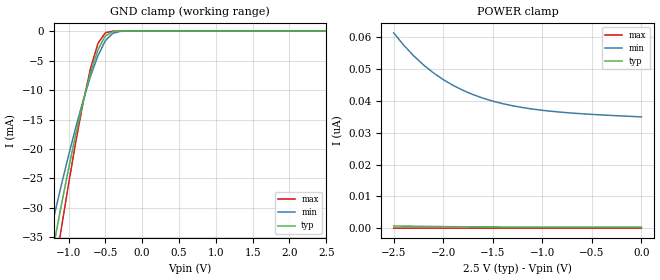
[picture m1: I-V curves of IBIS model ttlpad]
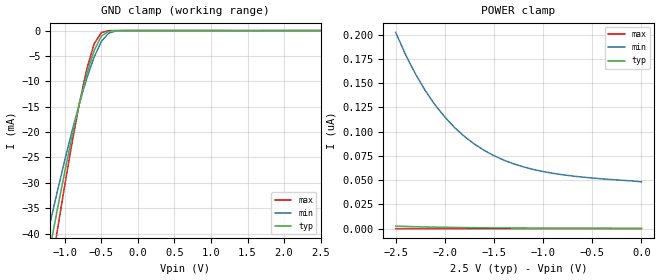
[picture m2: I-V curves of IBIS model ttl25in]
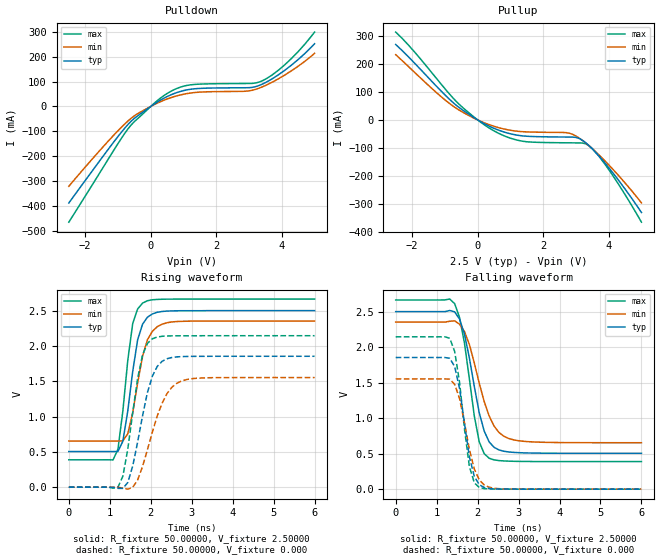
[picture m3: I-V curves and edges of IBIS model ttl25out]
| IBIS file idt45t9050.ibs created by s2ibis2 version 1.2
| North Carolina State University Electronics Research Laboratory  1995
[IBIS ver]   3.2
[File name]   idt45t9050.ibs
[File Rev]   1.0
[Date]   Friday, November 09, 2001
[Source]   Integrated Device Technology, Inc.
[Notes]
[Disclaimer] Integrated Device Technology, Inc. ("IDT") hereby grants the
   user of this IBIS model a non-exclusive, nontransferable
   license to use this IBIS model under the following terms. The
   user is granted this license only to use the IBIS model and is
   not granted rights to sell, copy (except as needed to run the
   IBIS model), rent, lease or sub-license the IBIS model in
   whole or in part, or in modified form to anyone. The User may
   modify the IBIS model to suit its specific applications, but
   rights to derivative works and such modifications shall belong
   to IDT. This IBIS model is provided on an AS IS" basis and IDT
   makes absolutely no warranty with respect to the information
   contained herein. IDT DISCLAIMS AND CUSTOMER WAIVES ALL
   WARRANTIES, EXPRESS AND IMPLIED, INCLUDING WARRANTIES OF
   MERCHANTABILITY AND FITNESS FOR A PARTICULAR PURPOSE. THE
   ENTIRE RISK AS TO QUALITY AND PERFORMANCE IS WITH THE USER
   ACCORDINGLY, IN NO EVENT SHALL IDT BE LIABLE FOR ANY DIRECT OR
   INDIRECT DAMAGES, WHETHER IN CONTRACT OR TORT, INCLUDING ANY
   LOST PROFITS OR OTHER INCIDENTAL, CONSEQUENTIAL, EXEMPLARY, OR
   PUNITIVE DAMAGES ARISING OUT OF THE USE OR APPLICATION OF THE
   IBIS model. Further, IDT reserves the right to make changes
   without notice to any product herein to improve reliability,
   function, or design. IDT does not convey any license under
   patent rights or any other intellectual property rights,
   including those of third parties. IDT is not obligated to
   provide maintenance or support for the licensed IBIS model.
[Copyright]   Copyright 2001, Integrated Device Technology, Inc. all rights
   reserved
|   Component idt45t9050
[Component]   idt45t9050
[Manufacturer]   Integrated Device Technology
|Package   PG28
[Package]
| variable   typ   min   max
R_pkg   2.40000m   2.40000m   2.40000m
L_pkg   0.90000nH   0.90000nH   0.90000nH
C_pkg   60.0000fF   60.0000fF   60.0000fF
[Pin]  signal_name   model_name   R_pin   L_pin   C_pin
1   GL   ttlpad
2   VDD   POWER
3   GND   GND
4   GX   ttlpad
5   VDDQ   POWER
6   Q1   ttl25out
7   GND   GND
8   A   ttl25in
9   Q5   ttl25out
10   VDDQ   POWER
11   GND   GND
12   VDD   POWER
13   VDD   POWER
14   NC   NC
15   NC   NC
16   VDDQ   POWER
17   GND   GND
18   GND   GND
19   VDDQ   POWER
20   Q4   ttl25out
21   Q3   ttl25out
22   GND   GND
23   Q2   ttl25out
24   VDDQ   POWER
25   GND   GND
26   GND   GND
27   VDDQ   POWER
28   GND   GND
[Pin Mapping]  pulldown_ref   pullup_ref   gnd_clamp_ref   power_clamp_ref
1   GND   VDD
2   NC   VDD
3   GND   NC
4   GND   VDD
5   NC   VDDQ
6   GND   VDDQ
7   GND   NC
8   GND   VDD
9   GND   VDDQ
10   NC   VDDQ
11   GND   NC
12   NC   VDD
13   NC   VDD
14   NC   NC
15   NC   NC
16   NC   VDDQ
17   GND   NC
18   GND   NC
19   NC   VDDQ
20   GND   VDDQ
21   GND   VDDQ
22   GND   NC
23   GND   VDDQ
24   NC   VDDQ
25   GND   NC
26   GND   NC
27   NC   VDDQ
28   GND   NC
| Models and submodels in the file (3): ttlpad (Input), ttl25in (Input), ttl25out (Output)
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|   Model ttlpad
[Model]   ttlpad
Model_type   Input
Polarity   Non-Inverting
Vinl =  0.70000V
Vinh =  1.70000V
Vmeas =  1.25000V
C_comp   5.00000pF   5.00000pF   5.00000pF
[Temperature Range]   45.00000   0.14000k   -30.00000
[Voltage Range]   2.50000V   2.30000V   2.70000V
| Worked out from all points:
|   GND clamp passes 1 mA (typ) near -0.51 V on its own axis
[GND_clamp]
| voltage   I(typ)   I(min)   I(max)
-2.5V     -129.2mA   -109.1mA   -150.6mA
-1.3V     -43.01mA   -37.08mA   -49.74mA
-1.2V     -36.24mA   -31.57mA   -41.59mA
-1.1V     -29.66mA   -26.23mA   -33.63mA
-900mV    -17.36mA   -16.23mA   -18.68mA
-800mV    -11.85mA   -11.7mA    -12mA
-700mV    -6.996mA   -7.615mA   -6.253mA
-600mV    -3.137mA   -4.151mA   -2.071mA
-500mV    -815.1uA   -1.634mA   -278.8uA
-400mV    -95.37uA   -373.7uA   -14.75uA
-300mV    -5.658uA   -48.78uA   -281.7nA
2.5V      324.7pA    35.28nA    828.2fA
[POWER_clamp]
| voltage   I(typ)   I(min)   I(max)
-2.5V     698.6pA    61.39nA    2.05pA
-2.4V     644.6pA    57.56nA    1.88pA
-2.3V     597.5pA    54.23nA    1.737pA
-2.2V     556.7pA    51.34nA    1.611pA
-2.1V     521.4pA    48.85nA    1.499pA
-1.9V     465pA      44.88nA    1.333pA
-1.8V     442.7pA    43.32nA    1.256pA
-1.6V     407.7pA    40.88nA    1.155pA
-1.3V     373.1pA    38.48nA    1.037pA
-1V       352.5pA    37.05nA    965.9fA
-600mV    337.2pA    35.97nA    899.5fA
0V        324.7pA    34.99nA    849.9fA
|   Model ttl25in
[Model]   ttl25in
Model_type   Input
Polarity   Non-Inverting
Vinl =  0.70000V
Vinh =  1.70000V
Vmeas =  1.25000V
C_comp   5.00000pF   5.00000pF   5.00000pF
[Temperature Range]   45.00000   0.14000k   -30.00000
[Voltage Range]   2.50000V   2.30000V   2.70000V
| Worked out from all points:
|   GND clamp passes 1 mA (typ) near -0.49 V on its own axis
[GND_clamp]
| voltage   I(typ)   I(min)   I(max)
-2.5V     -150.1mA   -128.5mA   -173mA
-1.3V     -50.47mA   -44.23mA   -57.51mA
-1.2V     -42.64mA   -37.76mA   -48.2mA
-1.1V     -35.02mA   -31.48mA   -39.1mA
-900mV    -20.73mA   -19.68mA   -21.96mA
-800mV    -14.28mA   -14.3mA    -14.26mA
-700mV    -8.553mA   -9.407mA   -7.567mA
-600mV    -3.939mA   -5.223mA   -2.609mA
-500mV    -1.074mA   -2.122mA   -375.8uA
-400mV    -131.3uA   -507.1uA   -20.31uA
-300mV    -7.825uA   -67.79uA   -384.6nA
2.5V      443.6pA    49.9nA     1.135pA
[POWER_clamp]
| voltage   I(typ)   I(min)   I(max)
-2.5V     2.616nA    202.4nA    8.153pA
-2.4V     2.294nA    179.5nA    7.17pA
-2.3V     2.014nA    159.7nA    6.305pA
-2.2V     1.772nA    142.5nA    5.573pA
-2.1V     1.564nA    127.7nA    4.925pA
-1.9V     1.231nA    104.2nA    3.911pA
-1.8V     1.1nA      95.05nA    3.496pA
-1.6V     895.6pA    80.73nA    2.854pA
-1.3V     696.3pA    66.86nA    2.22pA
-1V       581.4pA    58.89nA    1.825pA
-600mV    500.6pA    53.16nA    1.519pA
0V        443.6pA    48.28nA    1.265pA
|   Model ttl25out
[Model]   ttl25out
Model_type   Output
Polarity   Non-Inverting
Vmeas =  1.25000V
C_comp   5.00000pF   5.00000pF   5.00000pF
[Temperature Range]   45.00000   0.14000k   -30.00000
[Voltage Range]   2.50000V   2.30000V   2.70000V
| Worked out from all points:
|   slope of the pulldown table from 0 to 0.375 V, typ, clamps not added: 12.1 ohm
|   slope of the pullup table from 0 to 0.375 V, typ, clamps not added: 15.8 ohm
|   rising waveform, R_fixture 50.00000, V_fixture 2.50000: 20-80 % time 297ps typ, 346ps min, 268ps max; typ from 0.505 V to 2.5 V
|   rising waveform, R_fixture 50.00000, V_fixture 0.000: 20-80 % time 408ps typ, 515ps min, 338ps max; typ from 0 V to 1.85 V
|   falling waveform, R_fixture 50.00000, V_fixture 2.50000: 20-80 % time 412ps typ, 503ps min, 353ps max; typ from 2.5 V to 0.505 V
|   falling waveform, R_fixture 50.00000, V_fixture 0.000: 20-80 % time 301ps typ, 337ps min, 273ps max; typ from 1.85 V to 0 V
[Pulldown]
| voltage   I(typ)   I(min)   I(max)
-2.5V     -387.1mA   -320.1mA   -464mA
-1.3V     -172.3mA   -139.4mA   -211.9mA
-700mV    -73.11mA   -58.92mA   -90.86mA
-400mV    -37.65mA   -28.88mA   -48.96mA
300mV     25.63mA    19.24mA    33.79mA
700mV     51.07mA    38.83mA    66.42mA
1.1V      66.37mA    51.46mA    84.22mA
2.9V      74.99mA    61.06mA    92.02mA
3.4V      89.1mA     78.19mA    102.5mA
4.1V      145.9mA    126.7mA    168.2mA
4.5V      188.2mA    161.4mA    220mA
5V        251.4mA    212.9mA    298.1mA
[Pullup]
| voltage   I(typ)   I(min)   I(max)
-2.5V     269.9mA    233.5mA    314.3mA
-800mV    67.39mA    53.61mA    84.83mA
-300mV    22.62mA    17.64mA    28.64mA
400mV     -25.11mA   -19.06mA   -32.59mA
900mV     -46.72mA   -35.05mA   -61.28mA
1.4V      -57.66mA   -42.47mA   -76.9mA
2.8V      -61.54mA   -47.61mA   -82.16mA
3.1V      -66.62mA   -65.23mA   -82.46mA
3.4V      -92.17mA   -92.61mA   -92.89mA
3.7V      -128.7mA   -125.1mA   -129.7mA
4.1V      -185.6mA   -173.4mA   -194.7mA
5V        -331.7mA   -297.2mA   -366.3mA
[Ramp]
| variable   typ   min   max
dV/dt_r   1.11240/0.40540n   0.93180/0.51638n   1.28700/0.32701n
dV/dt_f   1.19718/0.40789n   1.02540/0.47741n   1.36518/0.35300n
R_load = 50.00000
[Rising Waveform]
R_fixture = 50.00000
V_fixture = 2.50000
C_fixture = 0.000F
R_dut = 2.40000m
L_dut = 0.90000nH
C_dut = 60.00000fF
| time   V(typ)   V(min)   V(max)
0s        504.8mV    653.9mV    388.4mV
1.08ns    504.7mV    653.9mV    386.6mV
1.2ns     506.3mV    653.7mV    539.2mV
1.32ns    652.2mV    656.5mV    1.083V
1.44ns    1.082V     757.3mV    1.799V
1.56ns    1.639V     1.056V     2.318V
1.8ns     2.308V     1.853V     2.607V
2.04ns    2.454V     2.208V     2.654V
2.4ns     2.494V     2.329V     2.663V
6ns       2.5V       2.353V     2.664V
[Rising Waveform]
R_fixture = 50.00000
V_fixture = 0.000
C_fixture = 0.000F
R_dut = 2.40000m
L_dut = 0.90000nH
C_dut = 60.00000fF
| time   V(typ)   V(min)   V(max)
0s        0V         0V         0V
1.2ns     -15.93mV   -14.73uV   745uV
1.32ns    -16.19mV   -13.53mV   156.8mV
1.44ns    66.38mV    -27.62mV   540.4mV
1.68ns    639mV      101.2mV    1.542V
1.8ns     1.011V     293.9mV    1.873V
2.04ns    1.573V     781.8mV    2.102V
2.4ns     1.819V     1.329V     2.142V
2.76ns    1.849V     1.506V     2.144V
6ns       1.854V     1.553V     2.145V
[Falling Waveform]
R_fixture = 50.00000
V_fixture = 2.50000
C_fixture = 0.000F
R_dut = 2.40000m
L_dut = 0.90000nH
C_dut = 60.00000fF
| time   V(typ)   V(min)   V(max)
0s        2.5V       2.353V     2.664V
1.44ns    2.497V     2.37V      2.612V
1.56ns    2.393V     2.322V     2.416V
1.68ns    2.18V      2.219V     2.054V
1.92ns    1.444V     1.774V     1.028V
2.04ns    1.075V     1.492V     666.2mV
2.28ns    667.3mV    1.033V     435.9mV
2.52ns    552.7mV    799.5mV    402.6mV
2.88ns    517.9mV    694.1mV    392.5mV
6ns       504.8mV    653.9mV    388.4mV
[Falling Waveform]
R_fixture = 50.00000
V_fixture = 0.000
C_fixture = 0.000F
R_dut = 2.40000m
L_dut = 0.90000nH
C_dut = 60.00000fF
| time   V(typ)   V(min)   V(max)
0s        1.854V     1.553V     2.145V
1.32ns    1.843V     1.548V     2.125V
1.44ns    1.728V     1.476V     1.939V
1.56ns    1.416V     1.274V     1.5V
1.68ns    923.4mV    932.4mV    843mV
1.8ns     451.6mV    556.4mV    314.5mV
1.92ns    177.3mV    281.9mV    89.2mV
2.04ns    63.41mV    130.8mV    24.09mV
2.52ns    2.361mV    6.883mV    945.9uV
6ns       679.4nV    2.744uV    0V
